FUNCTION_BLOCK FB_MachineData
VAR_INPUT
	bRunOnCeDevice				: BOOL	:= TRUE;	(*在CE系统运行*)
	sgFilePath					: STRING(255)	:= 'Data\Machine\';	(*文件路径*)
	sgFileName					: STRING(255)	:= 'Test';			(*文件名*)
	eFileType					: E_FileType	:= eFileType_XML;	(*文件类型, 只支持 eFileType_XML 和 eFileType_BIN 两种类型*)
(*参数和备份(用来比较参数是否修改的)的类型必须一致, 把两个变量的首地址和数据长度传到功能块*)
	pMacData					: PVOID;			(*配方首地址*)
	pBakData					: PVOID;			(*配方备份数据首地址, 数据类型必须和配方一样*)
	nMacSize					: UDINT;			(*配方的字节数*)
	tAutoSave					: TIME	:= T#10S;	(*配方改变后, 延时保存*)
END_VAR
VAR_OUTPUT
(*状态*)
	bInitialDone				: BOOL;	(*初始化完成*)
	bDone						: BOOL;
	bBusy						: BOOL;
	bError						: BOOL;
END_VAR
VAR		
	eStep						: INT;
(*Last status*)
	s_sLastExecuteResult		: ST_LastExecutionResult_File;
(*FB*)
	s_fbWriteReadFileXml		: FB_WriteReadFileXML_ByAddr;
	s_fbWriteReadFileBin		: FB_WriteReadFileBIN_2;
	s_nErrorCounter				: UDINT;
(*参数改变, 延时触发写文件*)
	s_tonDataChange				: TON;
	s_bDataChange				: BOOL;
	s_bManualWriteOnce			: BOOL;
	s_fbWriteReadFile: BOOL;
END_VAR

(*==================================================================
配置
==================================================================*)
	s_tonDataChange.PT					:= tAutoSave;		(*参数修改后, 延时写入临时文件(作用是掉电保持)的时间*)


(*==================================================================
变量地址是否有误
==================================================================*)
IF pMacData = 0 OR nMacSize <= 0 OR pBakData = 0 THEN
	bInitialDone := bBusy := bDone := FALSE;
	eStep := 0;
	bError := TRUE;
	RETURN;
END_IF


(*==================================================================
判断参数是否变化, 变化后, 延时写入文件
==================================================================*)
(*参数比较, 有变化时, 延时置位s_bDataChange, 将当前参数写到临时文件中*)
IF pMacData <> 0 AND nMacSize > 0 AND pBakData <> 0 THEN
	IF MEMCMP(pBakData, pMacData, nMacSize) <> 0 THEN
		s_tonDataChange(IN := FALSE);		(*重新计时*)
		s_tonDataChange(IN := bInitialDone);	(*上载配方后, 只复制参数, 不写入临时文件*)
		MEMCPY(pBakData, pMacData, nMacSize);	(*比较不同, 重新定时, 并把数据复制到局部变量*)
	END_IF
ELSE
	bInitialDone := FALSE;
END_IF

s_tonDataChange();

s_bDataChange := FALSE;
IF s_tonDataChange.Q THEN
	s_tonDataChange(IN := FALSE);
	s_bDataChange := TRUE;
END_IF


(*保存路径*)
CASE eFileType OF
	eFileType_BIN:
		IF bRunOnCeDevice THEN
			s_fbWriteReadFileBin.sgDeviceName	:= '\Hard disk\';
		ELSE
			s_fbWriteReadFileBin.sgDeviceName	:= 'C:\';
		END_IF
			s_fbWriteReadFileBin.sgFolderName	:= sgFilePath;
			s_fbWriteReadFileBin.sgNetId		:= '';
			s_fbWriteReadFileBin.sOption.bSameAddress_RW	:= FALSE;
			s_fbWriteReadFileBin.sOption.sBinHeader.bInused	:= FALSE;
	ELSE
		IF bRunOnCeDevice THEN
			s_fbWriteReadFileXml.sgFilePath	:= '\Hard disk\';
		ELSE
			s_fbWriteReadFileXml.sgFilePath	:= 'C:\';
		END_IF
			s_fbWriteReadFileXml.sgFilePath	:= F_CreatePath(s_fbWriteReadFileXml.sgFilePath, sgFilePath, '', '');
END_CASE

(*读写流程*)
CASE eStep OF
	0:
		bDone := bError := FALSE;
		IF NOT bInitialDone THEN
			MEMSET(ADR(s_sLastExecuteResult), 0, SIZEOF(s_sLastExecuteResult));
			s_fbWriteReadFileXml(bReadFile := FALSE, bWriteFile := FALSE);
			s_fbWriteReadFileBin(bReadFile := FALSE, bWriteFile := FALSE);
			CASE eFileType OF
				eFileType_BIN:
					eStep := 100;
				ELSE
					eStep := 150;
			END_CASE
		ELSE
			IF s_bDataChange					(*数据变化后, 延时写入*)
			OR s_bManualWriteOnce THEN			(*手动写入一次(测试用)*)
				MEMSET(ADR(s_sLastExecuteResult), 0, SIZEOF(s_sLastExecuteResult));
				s_bDataChange := FALSE;
				s_bManualWriteOnce := FALSE;
				s_fbWriteReadFileXml(bReadFile := FALSE, bWriteFile := FALSE);
				s_fbWriteReadFileBin(bReadFile := FALSE, bWriteFile := FALSE);
				CASE eFileType OF
					eFileType_BIN:
						eStep := 200;
					ELSE
						eStep := 250;
				END_CASE
			END_IF
		END_IF

	100:	(*读取BIN文件*)
		s_fbWriteReadFileBin.pDestBuffer	:= pMacData;
		s_fbWriteReadFileBin.u32DestSize	:= nMacSize;
		s_fbWriteReadFileBin.sgFileName		:= sgFileName;
		s_fbWriteReadFileBin(bReadFile := TRUE);
		s_nErrorCounter					:= 0;
		eStep := 110;
	110:
		s_fbWriteReadFileBin(bReadFile := TRUE);
		IF NOT s_fbWriteReadFileBin.bBusy THEN
			IF NOT s_fbWriteReadFileBin.bError THEN
				MEMCPY(pBakData, pMacData, nMacSize);	(*读取完, 把值传给中间变量*)
				bDone := TRUE;
				eStep := 0;
			ELSE
				s_nErrorCounter := s_nErrorCounter + 1;	(*连续读写失败, 可能是文件不存在, 跳过*)
				IF s_nErrorCounter > 5 THEN
					bError := TRUE;
					eStep := 0;
				END_IF
			END_IF
			s_bDataChange := FALSE;
			s_bManualWriteOnce := FALSE;
			s_fbWriteReadFileBin(bReadFile := FALSE, bWriteFile := FALSE);
		END_IF

	150:	(*读取XML文件*)
		s_fbWriteReadFileXml.pDataADR		:= pMacData;
		s_fbWriteReadFileXml.u32DataSIZEOF	:= nMacSize;
		s_fbWriteReadFileXml.sgFileName		:= sgFileName;
		s_fbWriteReadFileXml(bReadFile := TRUE);
		s_nErrorCounter					:= 0;
		eStep := 160;
	160:
		s_fbWriteReadFileXml(bReadFile := TRUE);
		IF NOT s_fbWriteReadFileXml.bBusy THEN
			IF NOT s_fbWriteReadFileXml.bError THEN
				MEMCPY(pBakData, pMacData, nMacSize);	(*读取完, 把值传给中间变量*)
				bDone := TRUE;
				eStep := 0;
			ELSE
				s_nErrorCounter := s_nErrorCounter + 1;	(*连续读写失败, 可能是文件不存在, 跳过*)
				IF s_nErrorCounter > 5 THEN
					bError := TRUE;
					eStep := 0;
				END_IF
			END_IF
			s_bDataChange := FALSE;
			s_bManualWriteOnce := FALSE;
			s_fbWriteReadFileXml(bReadFile := FALSE, bWriteFile := FALSE);
		END_IF

	200:	(*写入BIN文件*)
		s_fbWriteReadFileBin.pSrcBuffer		:= pMacData;
		s_fbWriteReadFileBin.u32SrcSize		:= nMacSize;
		s_fbWriteReadFileBin.sgFileName		:= sgFileName;
		s_fbWriteReadFileBin(bWriteFile := TRUE);
		eStep := 210;
	210:
		s_fbWriteReadFileBin(bWriteFile := TRUE);
		IF s_fbWriteReadFileBin.bWriteFile THEN
			s_fbWriteReadFileBin(bWriteFile := TRUE);
			IF NOT s_fbWriteReadFileBin.bBusy THEN
				IF NOT s_fbWriteReadFileBin.bError THEN
					bDone := TRUE;
				ELSE
					bError := TRUE;
				END_IF
				s_fbWriteReadFileBin(bReadFile := FALSE, bWriteFile := FALSE);
				eStep := 0;
			END_IF
		END_IF
	250:	(*写入XML文件*)
		s_fbWriteReadFileXml.pDataADR		:= pMacData;
		s_fbWriteReadFileXml.u32DataSIZEOF	:= nMacSize;
		s_fbWriteReadFileXml.sgFileName		:= sgFileName;
		s_fbWriteReadFileXml(bWriteFile := TRUE);
		eStep := 260;
	260:
		s_fbWriteReadFileXml(bWriteFile := TRUE);
		IF s_fbWriteReadFileXml.bWriteFile THEN
			s_fbWriteReadFileXml(bWriteFile := TRUE);
			IF NOT s_fbWriteReadFileXml.bBusy THEN
				IF NOT s_fbWriteReadFileXml.bError THEN
					bDone := TRUE;
				ELSE
					bError := TRUE;
				END_IF
				s_fbWriteReadFileXml(bReadFile := FALSE, bWriteFile := FALSE);
				eStep := 0;
			END_IF
		END_IF
END_CASE


IF eStep <> 0 THEN
	bBusy := TRUE;
ELSE
	IF bBusy THEN
		bBusy := FALSE;
		bInitialDone := TRUE;			(*不管有没有读取成功, 都认为初始化完成*)
		s_sLastExecuteResult.bDone := bDone;
		s_sLastExecuteResult.bError := bError;
	END_IF
END_IF

END_FUNCTION_BLOCK
